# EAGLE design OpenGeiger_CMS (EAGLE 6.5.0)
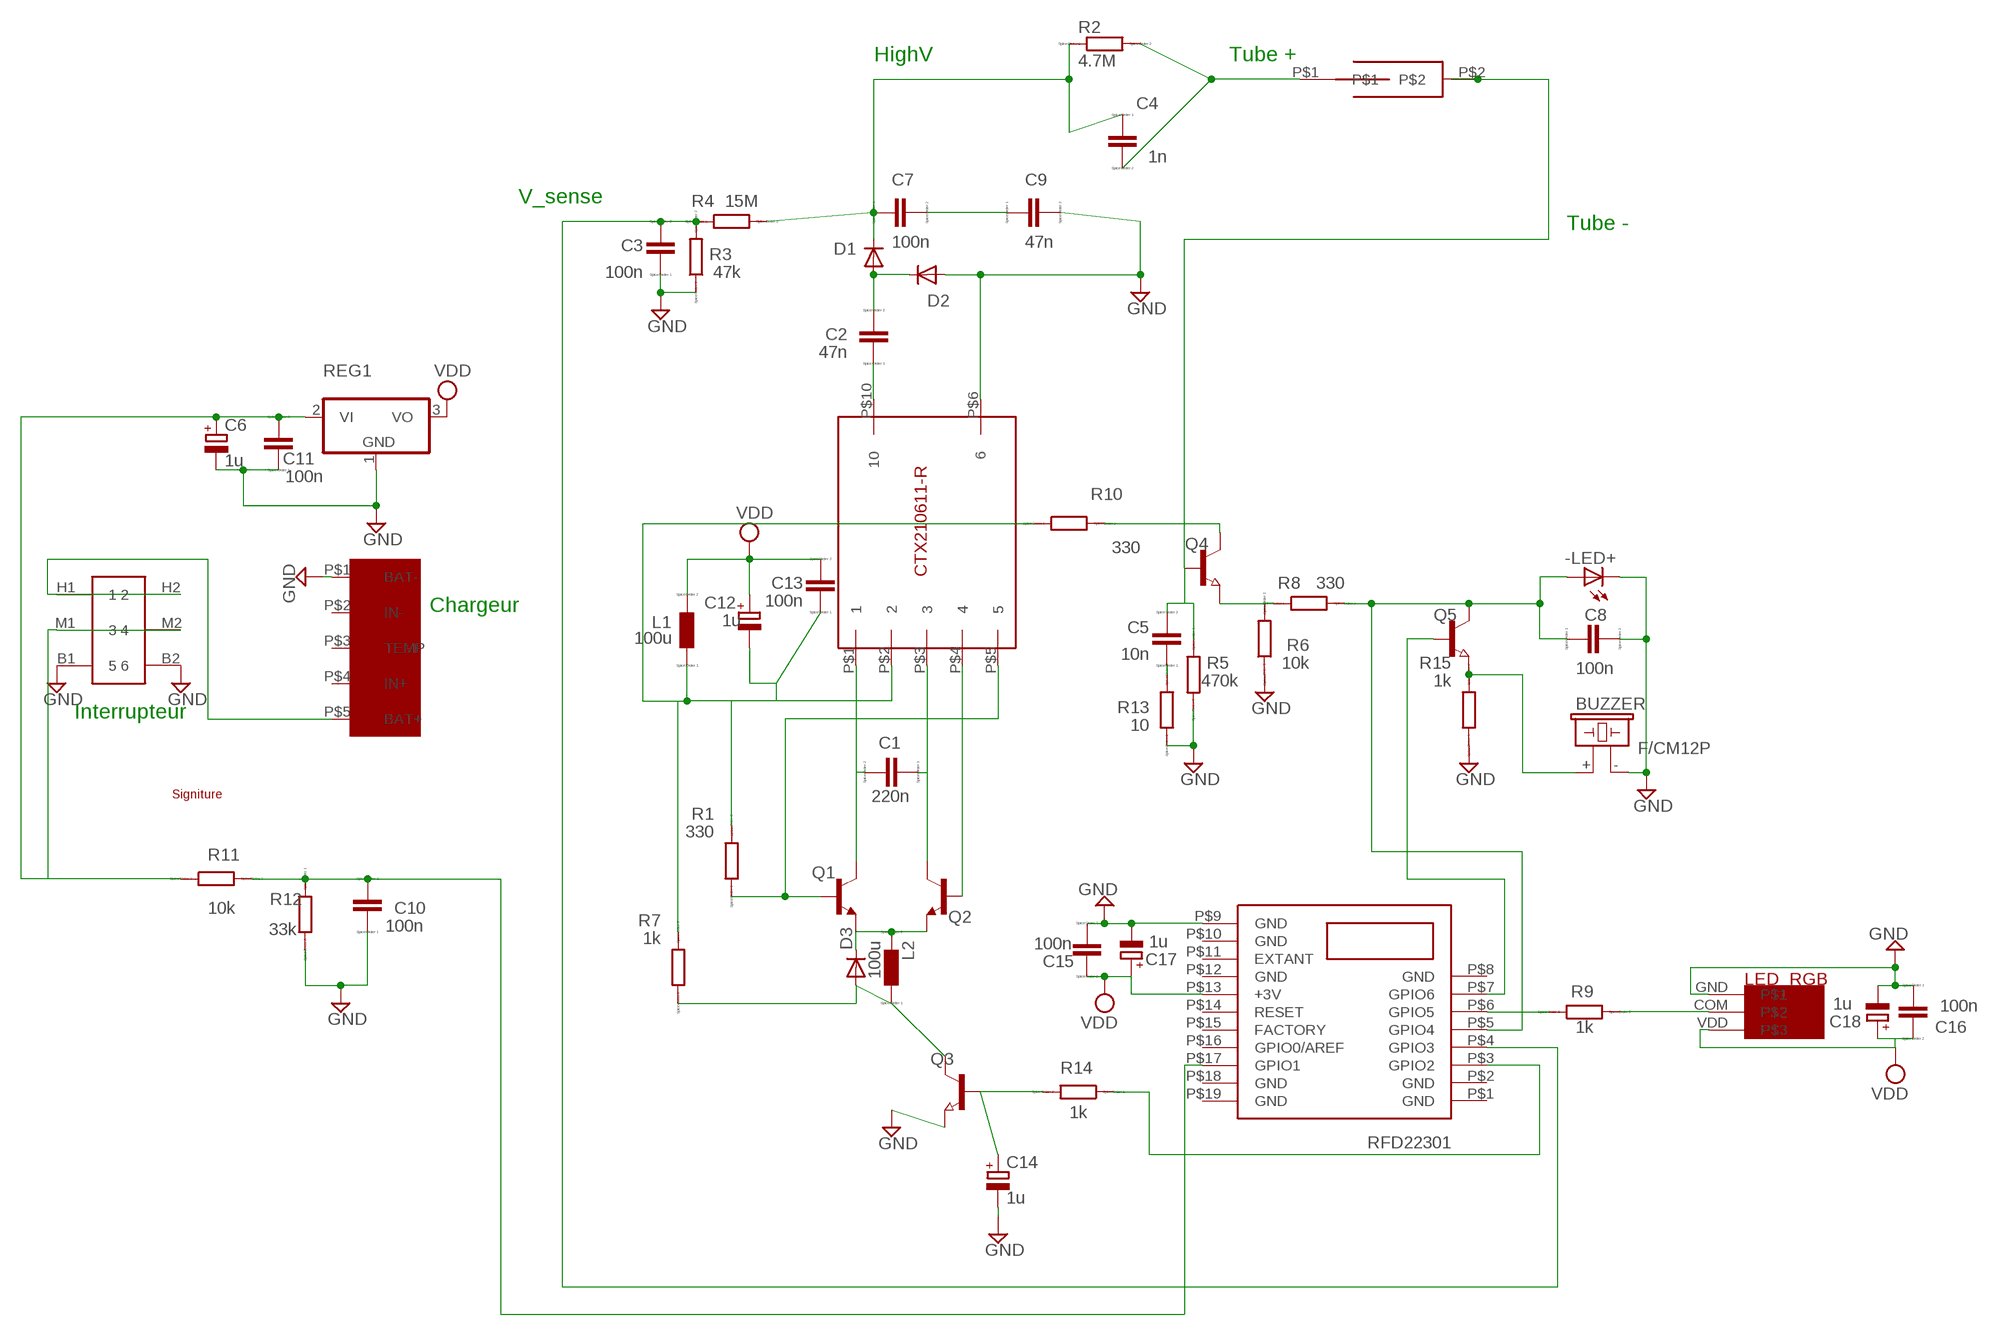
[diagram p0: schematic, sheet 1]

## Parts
-LED+  LEDIRL80A  [IRL80A]
BUZZER  F/CM12P  [F/CM12P]
C1  220n  CC0402  [C0402]
C2  47n  CC0402  [C0402]
C3  100n  CC0603  [C0603]
C4  1n  CC0603  [C0603]
C5  10n  CC0402  [C0402]
C6  1u  CPOL-EUB  [PANASONIC_B]
C7  100n  CC0603  [C0603]
C8  100n  CC0603  [C0603]
C9  47n  CC0402  [C0402]
C10  100n  CC0603  [C0603]
C11  100n  CC0603  [C0603]
C12  1u  CPOL-EUB  [PANASONIC_B]
C13  100n  CC0603  [C0603]
C14  1u  CPOL-EUB  [PANASONIC_B]
C15  100n  CC0603  [C0603]
C16  100n  CC0603  [C0603]
C17  1u  CPOL-EUB  [PANASONIC_B]
C18  1u  CPOL-EUB  [PANASONIC_B]
D1  DIODE-DO214AC  [DO214AC]
D2  DIODE-DO214AC  [DO214AC]
D3  DIODE-SOD123  [SOD123]
L1  100u  L  [L1812]
L2  100u  L  [L1812]
Q1  BC846  [SOT23]
Q2  BC846  [SOT23]
Q3  NPN-TRANSISTOR_SOT23  [SOT23]
Q4  BC337  NPN-TRANSISTOR_SOT23  [SOT23]
Q5  BC337  NPN-TRANSISTOR_SOT23  [SOT23]
R1  330  RR0603  [R0603]
R2  4.7M  RR0402  [R0402]
R3  47k  RR0402  [R0402]
R4  15M  RR0603  [R0603]
R5  470k  RR0402  [R0402]
R6  10k  RR0402  [R0402]
R7  1k  RR0402  [R0402]
R8  330  RR0603  [R0603]
R9  1k  RR0402  [R0402]
R10  330  RR0603  [R0603]
R11  10k  RR0402  [R0402]
R12  33k  RR0402  [R0402]
R13  10  RR0402  [R0402]
R14  1k  RR0402  [R0402]
R15  1k  RR0402  [R0402]
REG1  7812DT  [TO252]
RFD22301  RFD22301  [RFD22301]
U$1  CCFL_TRANSFO  [CCFL_TRANSFO]
U$2  TUBE  [TUBE]
U$3  LED_RGB  [LED_RGB]
U$4  INTERRUPTEUR  [INTERRUPTEUR]
U$5  ANTONYO  [ANTONYO]
U$6  CHARGEUR  [CHARGEUR]

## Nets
COUPS: -LED+.A C8.1 Q5.3(C) R8.2 RFD22301.P$5(GPIO4)
EMMETEUR_COMMUN: D3.C L2.2 Q1.2(E) Q2.2(E)
GND: -LED+.K(C) BUZZER.- C3.1 C6.- C8.2 C9.2 C10.1 C11.1 C14.- C15.1 C16.1 C17.- C18.- D2.A Q3.2(E) R3.1 R5.2 R6.1 R12.2 R13.1 R15.1 REG1.1(GND) RFD22301.P$9(GND) U$1.P$6 U$3.GND U$4.B1 U$4.B2 U$6.P$1(BAT-)
HIGH_V: C4.1 C7.1 D1.C R2.1 R4.2
N$2: C7.2 C9.1
N$3: C2.2 D1.A D2.C
N$4: Q1.1(B) R1.1 U$1.P$5
N$6: C5.2 Q4.1(B) R5.1 U$2.P$2
N$9: Q2.1(B) U$1.P$4
N$11: C5.1 R13.2
N$12: C4.2 R2.2 U$2.P$1
N$13: R9.1 RFD22301.P$6(GPIO5)
N$14: C10.2 R11.2 R12.1 RFD22301.P$17(GPIO1)
N$15: Q4.2(E) R6.2 R8.1
N$16: U$4.H1 U$4.H2 U$6.P$5(BAT+)
N$17: C1.2 Q1.3(C) U$1.P$1
N$18: C14.+ Q3.1(B) R14.2
N$19: Q4.3(C) R10.2
N$23: C1.1 Q2.3(C) U$1.P$3
N$27: Q5.1(B) RFD22301.P$7(GPIO6)
N$28: C2.1 U$1.P$10
N$32: R9.2 U$3.COM
N$38: BUZZER.+ Q5.2(E) R15.2
N$52: C6.+ C11.2 R11.1 REG1.2(VI) U$4.M1 U$4.M2
PWM: R14.1 RFD22301.P$3(GPIO2)
PWM_LISSé: D3.A L2.1 Q3.3(C) R7.1
V_SENSE: C3.2 R3.2 R4.1 RFD22301.P$4(GPIO3)
VDD: C12.+ C13.2 C15.2 C16.2 C17.+ C18.+ L1.2 REG1.3(VO) RFD22301.P$13(+3V) U$3.VDD
VDD_BOBINE: C12.- C13.1 L1.1 R1.2 R7.2 R10.1 U$1.P$2
Unconnected: RFD22301.P$1(GND) RFD22301.P$2(GND) RFD22301.P$8(GND) RFD22301.P$10(GND) RFD22301.P$11(EXTANT) RFD22301.P$12(GND) RFD22301.P$14(RESET) RFD22301.P$15(FACTORY) RFD22301.P$16(GPIO0/AREF) RFD22301.P$18(GND) RFD22301.P$19(GND) U$6.P$2(IN-) U$6.P$3(TEMP) U$6.P$4(IN+)

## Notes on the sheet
- HighV | Tube +
- V_sense
- Tube -
- Chargeur
- Interrupteur

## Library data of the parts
-LED+ = led:LED: LED
BUZZER = buzzer:F/CM12P: BUZZER; OC_FARNELL: unknown; OC_NEWARK: unknown
C1-C5 C7-C11 C13 C15 C16 = eagle-ltspice:C: CAPACITOR, European symbol; SPICEMODEL: NONE; SPICEPREFIX: C
C6 C12 C14 C17 C18 = rcl:CPOL-EU: POLARIZED CAPACITOR, European symbol
D1-D3 = diode:DIODE-: DIODE
L1 L2 = eagle-ltspice:L: INDUCTOR, European symbol; SPICEMODEL: NONE; SPICEPREFIX: L
Q1 Q2 = transistor:BC846: NPN TRANSISTOR
Q3-Q5 = semicon-smd-ipc:NPN-TRANSISTOR_: NPN TRANSISTOR
R1-R15 = eagle-ltspice:R: RESISTOR, European symbol; SPICEMODEL: NONE; SPICEPREFIX: R
REG1 = linear:78*: Positive VOLTAGE REGULATOR Source: http://cache.national.com/ds/LM/LM78L05.pdf http://www.fairchildsemi.com/ds/LM/LM7805.pdf
RFD22301 = RFDuino:RFD22301
U$1 = openGeiger:CCFL_TRANSFO
U$2 = openGeiger:TUBE
U$3 = openGeiger:LED_RGB
U$4 = openGeiger:INTERRUPTEUR
U$5 = openGeiger:ANTONYO
U$6 = openGeiger:CHARGEUR

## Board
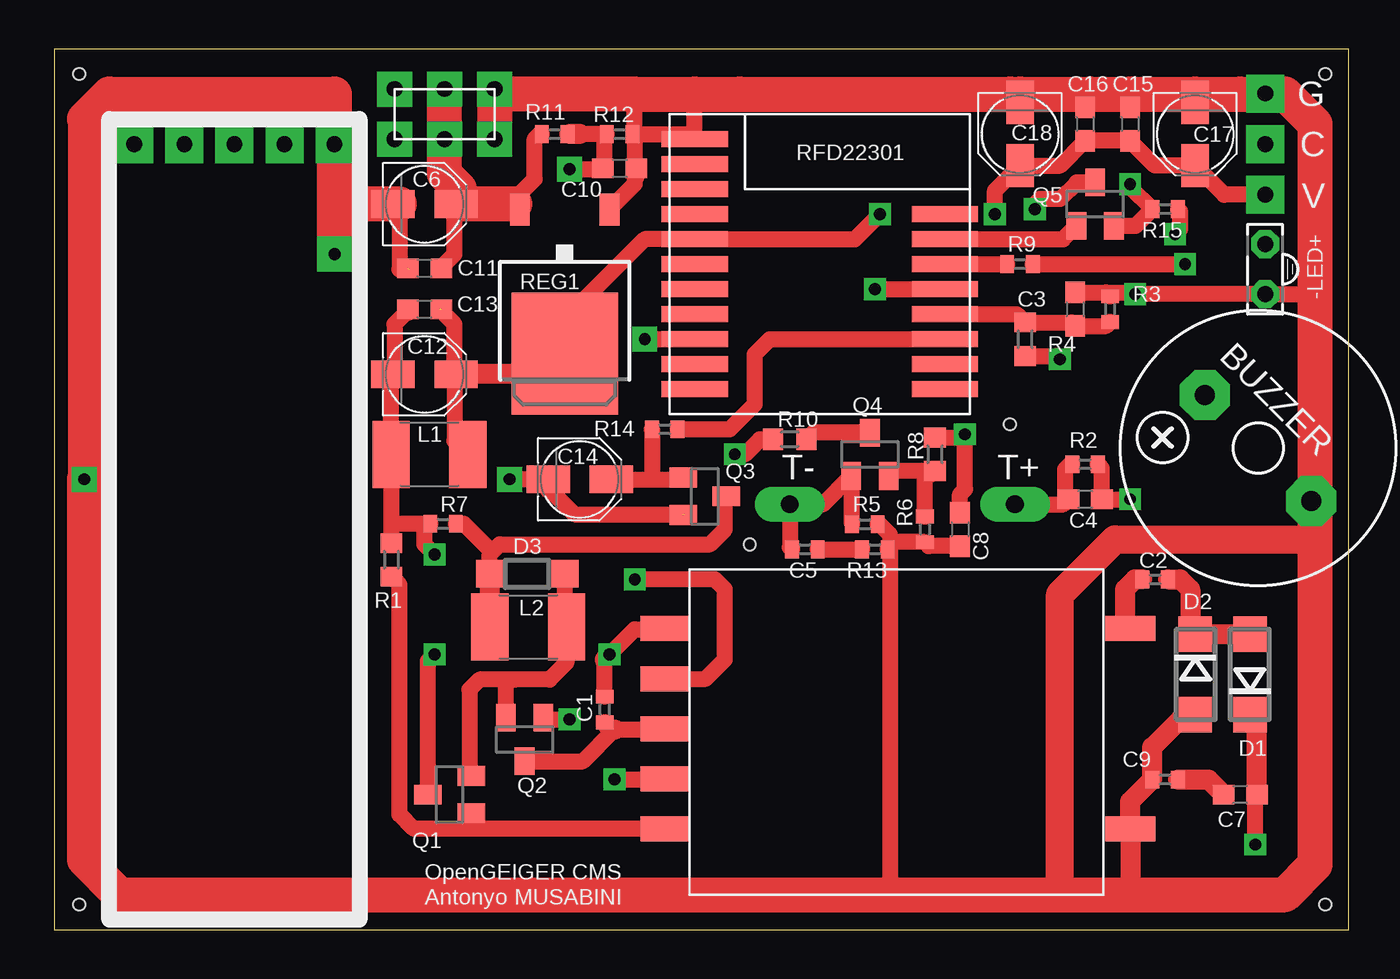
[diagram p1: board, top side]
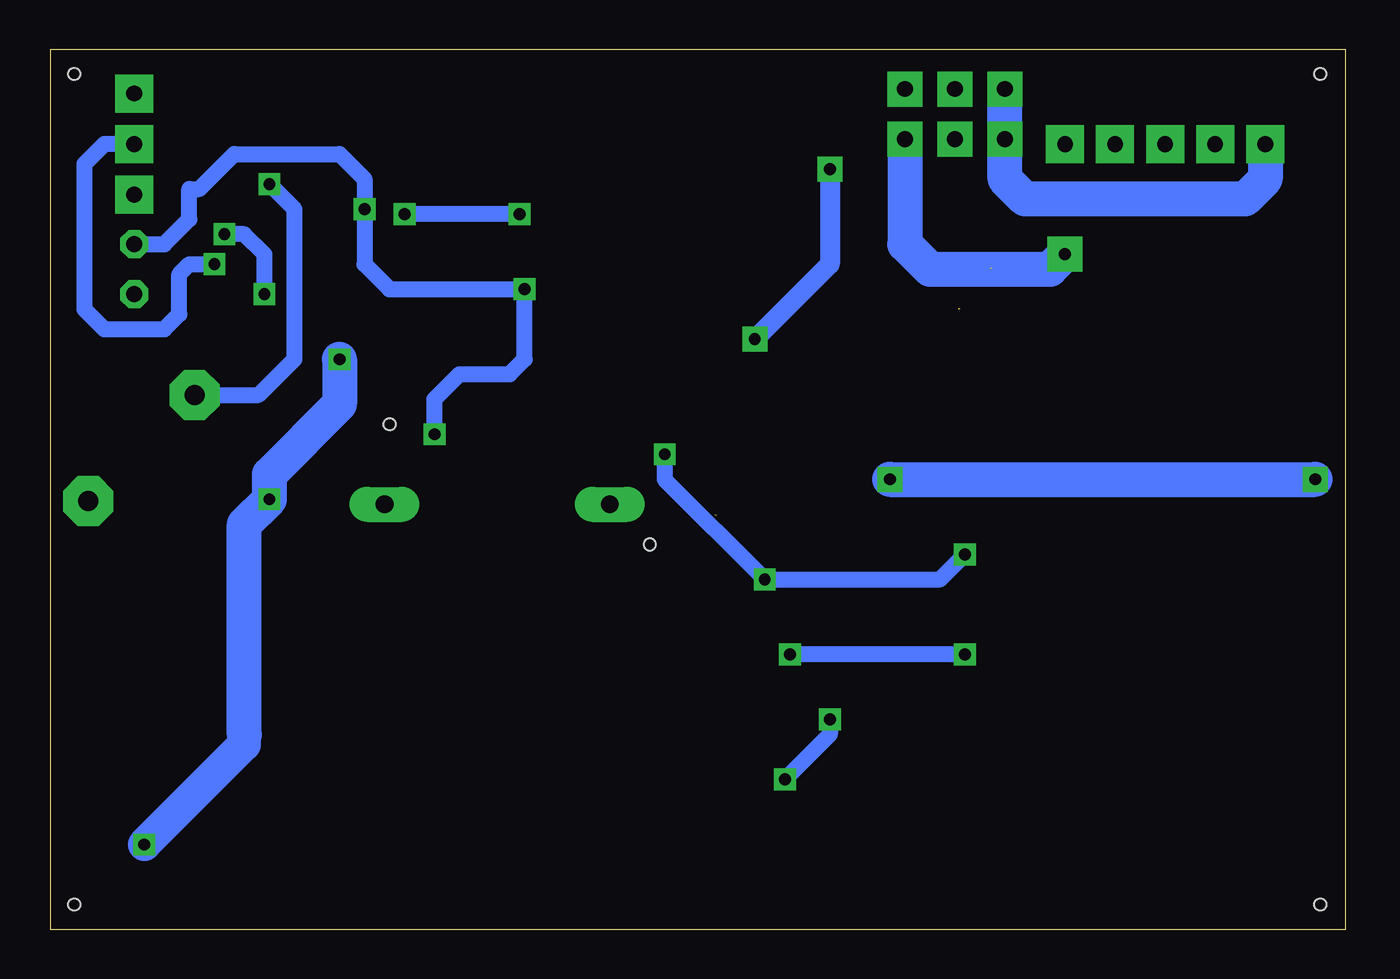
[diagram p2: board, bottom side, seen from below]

Size 65.71 x 44.69 mm. Coordinates in mm from the lower left corner, seen from the top.
Outline: 0,0 65.71,0 65.71,44.69 0,44.69 0,0
Copper layers (1*16): Top 0.035mm / dielectric 1.5mm / Bottom 0.035mm
Design rules "8mils": minimum track width 8mil, minimum drill 20mil, track to track 8mil, track to pad 8mil, pad to pad 8mil, via to via 8mil, smd to smd 8mil, copper to edge 10mil, drill to drill 8mil, minimum pad ring 12mil, minimum via ring 10mil, stop-mask expansion 4mil, vias tented up to drill 25mil, thermal gap 10mil
Holes 0.6 mm at 1.27,1.27 64.52,1.27 64.52,43.43 1.27,43.43 48.51,25.65 35.31,19.56

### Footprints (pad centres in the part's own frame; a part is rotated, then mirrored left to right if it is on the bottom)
IRL80A = drill 0.813 octagon: A 0,-1.27; K 0,1.27
F/CM12P = drill 1.016 pad 2.54 octagon: + 3.81,0; - -3.81,0
C0402 = smd 0.7 x 0.9: 1 -0.65,0; 2 0.65,0
C0603 = smd 1.1 x 1: 1 -0.85,0; 2 0.85,0
PANASONIC_B = smd 2.2 x 1.4: + 1.6,0; - -1.6,0
DO214AC = smd 1.8 x 1.7: A 2.05,0; C -2.05,0
SOD123 = smd 1.4 x 1.4: A 1.9,0; C -1.9,0
L1812 = smd 1.9 x 3.4: 1 -1.95,0; 2 1.95,0
SOT23 = smd 1 x 1.4: 1 -0.95,-1.1; 2 0.95,-1.1; 3 0,1.1
R0603 = smd 1 x 1.1: 1 -0.85,0; 2 0.85,0
R0402 = smd 0.7 x 0.9: 1 -0.65,0; 2 0.65,0
TO252 = smd 1 x 1.6: 1 -2.28,-4.8; 2 2.28,-4.8 | smd 5.4 x 6.2: 3 0,2.5
RFD22301 = smd 3.353 x 0.813: P$1 -6.35,6.35; P$2 -6.35,5.08; P$3 -6.35,3.81; P$4 -6.35,2.54; P$5 -6.35,1.27; P$6 -6.35,0; P$7 -6.35,-1.27; P$8 -6.35,-2.54; P$9 6.35,-6.35; P$10 6.35,-5.08; P$11 6.35,-3.81; P$12 6.35,-2.54; P$13 6.35,-1.27; P$14 6.35,0; P$15 6.35,1.27; P$16 6.35,2.54; P$17 6.35,3.81; P$18 6.35,5.08; P$19 6.35,6.35
CCFL_TRANSFO = smd 2.54 x 1.27: P$1 -1.238,13.5; P$2 -1.238,10.96; P$3 -1.238,8.42; P$4 -1.238,5.88; P$5 -1.238,3.34; P$6 22.365,3.34; P$10 22.365,13.5
TUBE = drill 0.9 pad 1.778 long: P$1 0,0; P$2 11.43,0
LED_RGB = drill 0.8 pad 1.93 square: COM 0,0; GND 0,2.57; VDD 0,-2.57
INTERRUPTEUR = drill 0.8 pad 1.778 square: B1 0,-5.08; B2 2.54,-5.08; H1 0,0; H2 2.54,0; M1 0,-2.54; M2 2.54,-2.54
CHARGEUR = drill 0.8 pad 1.93 square: P$1 0,0; P$2 0,-2.54; P$3 0,-5.08; P$4 0,-7.62; P$5 0,-10.16

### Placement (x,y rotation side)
-LED+  61.47,33.53 180 top
BUZZER  61.11,24.45 135 top
C1  27.94,11.18 90 top
C2  55.88,17.78 0 top
C3  51.82,31.5 270 top
C4  52.32,21.84 180 top
C5  38.1,19.3 180 top
C6  18.8,36.83 0 top
C7  60.2,6.86 180 top
C8  45.97,20.32 270 top
C9  56.39,7.62 180 top
C10  28.7,38.64 180 top
C11  18.8,33.57 0 top
C12  18.8,28.19 0 top
C13  18.8,31.5 0 top
C14  26.67,22.86 0 top
C15  54.61,40.89 270 top
C16  52.32,40.89 270 top
C17  57.91,40.39 270 top
C18  49.02,40.39 270 top
D1  60.71,12.95 90 top
D2  57.91,12.95 270 top
D3  24,18.06 180 top
L1  19.05,24.13 0 top
L2  24.05,15.37 0 top
Q1  20.07,6.86 90 top
Q2  23.88,9.65 180 top
Q3  33.02,22 270 top
Q4  41.4,24.13 0 top
Q5  52.83,36.83 0 top
R1  17.12,18.77 90 top
R2  52.32,23.62 180 top
R3  53.59,31.5 270 top
R4  49.28,29.97 270 top
R5  41.15,20.57 0 top
R6  44.2,20.32 90 top
R7  19.74,20.6 180 top
R8  44.7,24.13 90 top
R9  49.02,33.78 0 top
R10  37.34,24.89 0 top
R11  25.4,40.39 0 top
R12  28.7,40.39 0 top
R13  41.66,19.3 180 top
R14  30.99,25.4 180 top
R15  56.39,36.58 180 top
REG1  25.91,31.75 180 top
RFD22301  38.86,33.78 180 top
U$1  32.26,1.78 0 top
U$2  48.77,21.59 180 top
U$3  61.47,39.88 0 top
U$4  17.27,40.13 90 top
U$5  18.8,1.27 0 top
U$6  14.22,39.88 270 top

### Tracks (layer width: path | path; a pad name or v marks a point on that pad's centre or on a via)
COUPS  (via drill 0.6 pad 1.02)
  Top 0.813: 45.72,32.51 RFD22301.P$5 v41.66,32.51 | R8.2 46.06,24.98 v46.23,25.15 46.23,22.35 45.97,22.1 C8.1 | Q5.3 51.9,37.93 51.05,37.08 50.04,37.08 49.78,36.83 v49.78,36.58
  Bottom 0.813: v46.23,25.15 46.23,26.92 44.96,28.19 42.42,28.19 41.66,28.96 v41.66,32.51 48.51,32.51 49.78,33.78 v49.78,36.58 49.78,38.1 51.05,39.37 56.39,39.37 58.17,37.59 58.67,37.59 58.67,36.07 59.94,34.8 -LED+.A
EMMETEUR_COMMUN
  Top 0.813: 23.37,12.7 25.15,12.7 26,13.56 L2.2 25.9,15.47 D3.C | 23.37,12.7 21.59,12.7 21.08,12.19 21.08,7.89 Q1.2 | Q2.2 22.93,12.63 23.37,12.7
GND  (via drill 0.6 pad 1.02, 0.6 pad 1.27, 0.6 pad 1.78)  (2 unrouted)
  Top 0.254: R12.2 29.21,40.64 29.46,40.64 | 22.86,42.42 22.86,41.91 U$4.B2 | REG1.1 27.94,36.83 28.19,36.58 | 25.4,22.86 25.15,22.86 | 17.78,36.83 17.53,36.83
  Top 0.813: RFD22301.P$9 32.51,40.39 | 32.51,40.39 32.51,42.42 | 29.46,40.39 32.51,40.39 | 29.46,40.39 29.46,40.64 29.46,42.42 | 60.2,42.42 60.2,42.67 | 41.15,42.67 35.05,42.67 34.8,42.42 | 48.26,42.16 48.51,42.42 | 62.23,42.42 64.01,40.64 | 64.01,37.85 64.01,37.34 63.75,37.08 | 16.51,36.83 C6.- | 17.53,36.83 17.53,33.53 18.03,33.53 | 29.46,40.39 29.46,38.1 | 29.46,38.1 29.46,37.85 28.19,36.58 | 25.15,22.86 C14.- v23.11,22.86 | 25.15,22.35 26.42,21.08 32,21.08 | C18.- 49.02,42.42 | C16.1 52.32,42.16 52.58,42.42 | C15.1 54.61,42.42 | C17.- 57.91,42.42 | C3.1 53.39,32.35 | 53.39,32.35 R3.1 | 53.39,32.35 54.78,32.35 v54.86,32.26 -LED+.K 64.01,32.26 | v56.9,35.31 57.15,35.56 57.15,36.46 R15.1 | R5.2 41.91,20.57 42.42,20.07 42.42,19.42 | 42.42,19.42 R13.1 42.67,19.67 R6.1 44.4,19.47 C8.2 | 42.42,19.42 42.42,1.78 | BUZZER.- 63.8,19.86 63.75,19.81 | U$3.GND 62.45,42.45 62.74,42.16 | C10.1 29.55,38.18 29.46,38.1
  Top 1.016: 25.15,22.86 25.15,22.35 | 54.86,1.78 54.62,2.02 U$1.P$6 54.62,6.5 C9.2 55.74,9.26 57.15,10.67 57.68,10.67 D2.A
  Top 1.422: 51.05,2.03 51.05,17.02 53.85,19.81 63.75,19.81 64.01,19.81
  Top 1.676: 1.52,41.15 1.52,22.35
  Top 1.778: 1.52,41.15 2.79,42.42 14.22,42.42 U$6.P$1 | v1.52,22.86 1.52,22.35 1.52,3.56 3.3,1.78 42.42,1.78 54.86,1.78 62.48,1.78 64.01,3.3 64.01,19.81 64.01,32.26 64.01,37.85 64.01,40.64 64.01,40.89 62.74,42.16 62.48,42.42 60.2,42.42 57.91,42.42 54.61,42.42 52.58,42.42 49.02,42.42 48.51,42.42 34.8,42.42 32.51,42.42 29.46,42.42 22.86,42.42 22.35,42.42 U$4.B1 | U$6.P$1 14.22,39.12 | v14.22,34.29 14.22,36.83 | 14.22,36.83 U$6.P$1 | 17.53,36.83 C6.- 14.22,36.83
  Bottom 0.813: v54.86,32.26 54.86,34.29 55.88,35.31 v56.9,35.31
  Bottom 1.778: v23.11,22.86 v1.52,22.86 | 22.35,39.88 22.35,34.8 21.08,33.53 14.99,33.53 v14.22,34.29
HIGH_V  (via drill 0.6 pad 1.02)
  Top 0.813: R2.1 53.17,23.42 C4.1 v54.61,21.84 | R4.2 50.89,29.12 v51.05,28.96 | v60.96,4.32 60.96,6.77 C7.1
  Top 1.016: C7.1 61.05,10.56 D1.C
  Bottom 1.676: 55.88,9.91 55.88,9.4 v60.96,4.32
  Bottom 1.778: v51.05,28.96 51.05,26.67 54.61,23.11 v54.61,21.84 55.88,20.57 55.88,9.91
N$2
  Top 1.016: C9.1 58.59,7.62 C7.2
N$3
  Top 1.016: C2.2 57.15,17.78 57.66,17.27 57.66,15.26 D2.C D1.A
N$4
  Top 0.813: U$1.P$5 21.08,5.12 | 21.08,5.12 18.25,5.12 17.53,5.84 17.53,17.51 R1.1 | Q1.1 21.17,5.2 21.08,5.12
N$6
  Top 0.813: C5.2 37.34,19.42 U$2.P$2 39.01,21.59 Q4.1 40.5,22.98 R5.1
N$9  (via drill 0.6 pad 1.02)
  Top 0.813: Q2.1 24.83,10.73 24.89,10.67 v26.16,10.67 | v28.45,7.62 30.98,7.62 U$1.P$4
  Bottom 0.813: v26.16,10.67 26.16,9.91 v28.45,7.62
N$11
  Top 0.813: C5.1 R13.2
N$12
  Top 0.813: R2.2 51.56,23.62 51.31,23.37 51.31,22.01 C4.2 51.22,21.59 U$2.P$1
N$13
  Top 0.813: RFD22301.P$6 R9.1
N$14  (via drill 0.6 pad 1.27)
  Top 0.813: v26.16,38.61 27.85,38.61 | 27.94,40.39 26.67,40.39 R11.2 | 27.94,40.39 27.94,38.61 27.85,38.61 | v29.97,29.97 RFD22301.P$17 | 27.94,40.39 R12.1 | 27.85,38.61 C10.2
  Top 1.016: 26.67,40.39 26.16,40.39
  Bottom 1.016: v26.16,38.61 26.16,33.78 v29.97,29.97
N$15
  Top 0.813: R6.2 44.2,23.11 44.54,23.11 R8.1 42.6,23.28 Q4.2
N$16
  Bottom 1.778: U$6.P$5 4.06,38.1 5.08,37.08 16.26,37.08 17.27,38.1 U$4.H1 U$4.H2
N$17  (via drill 0.6 pad 1.02)
  Top 0.813: C1.2 27.94,13.72 | v28.19,13.97 29.46,15.24 30.98,15.24 | Q1.3 18.97,13.63 v19.3,13.97
  Top 1.016: 27.94,13.72 v28.19,13.97 | 30.98,15.24 U$1.P$1
  Bottom 0.813: v19.3,13.97 v28.19,13.97
N$18
  Top 0.813: C14.+ 30.23,22.86 | 30.23,22.86 31.83,22.86 Q3.1 | R14.2 30.34,22.97 30.23,22.86
N$19
  Top 0.813: Q4.3 38.53,25.23 R10.2
N$23
  Top 0.813: C1.1 27.94,10.41 28.19,10.16 | 30.98,10.16 28.45,10.16 26.84,8.55 Q2.3
  Top 1.016: 28.19,10.16 28.45,10.16 | 30.98,10.16 U$1.P$3
N$27
  Top 0.813: RFD22301.P$7 51.2,35.05 Q5.1
N$28
  Top 1.016: C2.1 54.86,17.78 54.36,17.27 54.36,15.54 U$1.P$10
N$32  (via drill 0.6 pad 1.02)
  Top 0.813: R9.2 v57.4,33.78
  Bottom 0.813: U$3.COM 62.99,39.88 64.01,38.86 64.01,31.5 62.99,30.48 59.94,30.48 59.18,31.24 59.18,33.27 58.67,33.78 v57.4,33.78
N$38  (via drill 0.6 pad 1.02)
  Top 0.813: Q5.2 54.89,35.73 R15.2 54.61,37.7 v54.61,37.85
  Bottom 0.813: BUZZER.+ 55.16,27.14 53.34,28.96 53.34,36.58 v54.61,37.85
N$52
  Top 0.813: 23.37,37.08 24.38,38.1 24.38,40.13 24.64,40.39 R11.1 | 20.32,36.58 20.32,34.29 19.56,33.53 19.56,33.57 C11.2 | 20.57,36.83 C6.+ | REG1.2 22.86,36.55 22.86,36.83
  Top 1.016: 23.37,36.83 23.37,37.08 | 20.32,36.58 20.57,36.83
  Top 1.778: 23.37,36.83 22.86,36.83 20.57,36.83 20.57,37.59 19.81,38.35 U$4.M1 U$4.M2
PWM
  Top 0.813: R14.1 34.29,25.4 35.56,26.67 35.56,29.21 36.32,29.97 RFD22301.P$3
PWM_LISSé
  Top 0.813: D3.A 22.1,19.05 22.23,19.18 | 22.23,19.18 22.61,19.56 33.27,19.56 34.04,20.32 34.04,21.91 | R7.1 20.8,20.6 22.23,19.18
  Top 1.016: L2.1 D3.A | 34.04,21.91 Q3.3
V_SENSE
  Top 0.813: RFD22301.P$4 48.86,31.24 R4.1 51.64,30.82 C3.2 53.39,30.65 R3.2
VDD  (via drill 0.6 pad 1.02)  (1 unrouted)
  Top 0.254: 20.32,27.94 C12.+ | 25.65,28.96 25.4,29.21 REG1.3
  Top 0.813: 25.91,30.99 29.97,35.05 RFD22301.P$13 40.64,35.05 v41.91,36.32 | 19.56,31.5 20.32,30.73 20.32,28.19 20.32,27.94 20.32,24.81 L1.2 | v47.75,36.32 47.75,37.52 C18.+ 51.07,38.79 C16.2 C15.2 55.87,38.79 C17.+ 59.39,37.31 U$3.VDD
  Top 1.016: 25.91,30.99 REG1.3 25.91,29.21 25.65,28.96 24.89,28.19 C12.+ 20.32,28.19
  Bottom 0.813: v41.91,36.32 v47.75,36.32
VDD_BOBINE  (via drill 0.6 pad 1.02)
  Top 0.813: 17.95,31.41 17.27,30.73 17.27,28.27 | L1.1 17.1,28.1 | R1.2 17.12,20.83 | 17.12,20.83 17.12,24.11 | 17.12,20.83 17.35,20.6 R7.2 18.8,20.31 18.8,19.56 v19.3,19.05 | U$1.P$2 33.06,12.74 34.04,13.72 34.04,17.27 33.53,17.78 v29.46,17.78 | R10.1 35.81,24.89 35.05,24.13 v34.54,24.13
  Top 1.016: C13.1 17.95,31.41 | 17.27,28.27 C12.- 17.1,28.1 | 17.12,24.11 L1.1
  Bottom 0.813: v19.3,19.05 20.57,17.78 v29.46,17.78 34.54,22.86 v34.54,24.13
